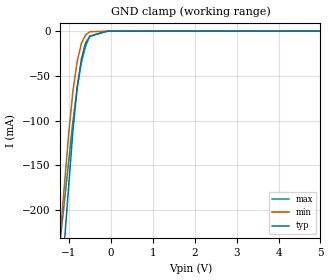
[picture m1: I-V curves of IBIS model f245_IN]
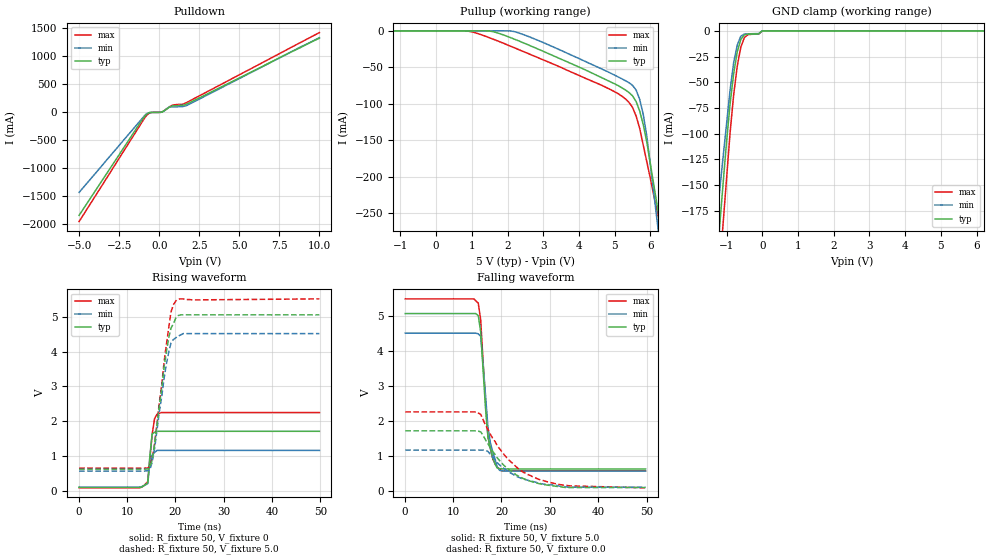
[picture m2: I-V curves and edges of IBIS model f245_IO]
| TEXAS INSTRUMENTS INCORPORATED
| Standard Linear and Logic Group
| IBIS Model of SN74F245
| OCTAL BUS TRANSCEIVERS WITH 3-STATE OUTPUTS
| SOIC 20-pin (DW), SOP 20-pin (NS), SSOP 20-pin (DB), P-DIP 20-pin (N)
[IBIS Ver]   3.2
[Comment Char]  |_char
[File Name]   sn74f245.ibs
[File Rev]   2.1 I_die
[Date]   Nov. 04, 2004
[Source]   File originated at Texas Instruments, Inc.
[Notes]   The following is a sample IBIS file for the F245.
   - FILE REV HISTORY
   - 2.1 Re-Release IBIS file on 11/05/04
   - Power-clamp data deleted as there is no power-clamp diode.
|   - All test data contained in this file are derived from
|   actual measurements.
|   - File created by Nobuhisa Ohtsubo, SLL Product Engineering.
[Disclaimer] Property of Texas Instruments Incorporated.  Unauthorized
   reproduction and/or distribution is strictly prohibited.
   This product is protected under copyright law.
   Created 2000, (C) Copyright 2000, Texas Instruments Inc.,
   All Rights Reserved.
   UNLESS THERE IS A SIGNED, WRITTEN AGREEMENT TO THE
   CONTRARY, TEXAS INSTRUMENTS () IS PROVIDING THE IBIS
   MODELS  AND WITHOUT ANY WARRANTY, EXPRESSED OR
   IMPLIED.  TI assumes no liability for:
   1) the accuracy of the IBIS models provided to your
   company;
   2) the proper functioning of these IBIS Models in your
   design or for any resulting applications; or
   3) infringement of patents, copyrights or intellectual
   property rights resulting from your use of these IBIS
   models.
   TI provides IBIS Models as a service to our customers.
   You and your company shall not distribute, sell or give
   these models to anyone else without prior written
   permission from TI.
   TI reserves the right to make changes to our products or
   to discontinue any semiconductor product or service
   without notice, and advises our customers to obtain the
   latest version of relevant information to verify, before
   placing orders, that the information being relied on is
   current.
   Please be aware that your receipt and use of the IBIS
   information provided shall serve as acceptance of these
   terms and conditions.  If you do not accept these terms,
   you should return or destroy the IBIS models and any
   other accompanying information immediately.
|   Component F245_DW
[Component]   f245_DW
[Manufacturer]  Texas Instruments, Inc.
[Package]
|   typ   min   max
R_pkg   0.038   0.033   0.045
L_pkg   5.012nH   4.110nH   6.349nH
C_pkg   0.717pF   0.530pF   0.868pF
[Pin]   signal_name   model_name   R_pin   L_pin   C_pin
1   DIR   f245_IN   0.058   5.115nH   0.725pF
2   A1   f245_IO   0.053   4.591nH   0.724pF
3   A2   f245_IO   0.049   3.754nH   0.572pF
4   A3   f245_IO   0.029   2.549nH   0.388pF
5   A4   f245_IO   0.031   2.317nH   0.316pF
6   A5   f245_IO   0.031   2.317nH   0.316pF
7   A6   f245_IO   0.029   2.556nH   0.399pF
8   A7   f245_IO   0.049   3.754nH   0.579pF
9   A8   f245_IO   0.053   4.591nH   0.724pF
10   GND   GND   0.058   5.115nH   0.725pF
11   B8   f245_IO   0.058   5.115nH   0.725pF
12   B7   f245_IO   0.053   4.591nH   0.724pF
13   B6   f245_IO   0.049   3.754nH   0.579pF
14   B5   f245_IO   0.029   2.557nH   0.399pF
15   B4   f245_IO   0.031   2.317nH   0.316pF
16   B3   f245_IO   0.031   2.317nH   0.316pF
17   B2   f245_IO   0.029   2.557nH   0.399pF
18   B1   f245_IO   0.049   3.754nH   0.579pF
19   OE_NOT   f245_IN   0.053   4.591nH   0.724pF
20   VCC   POWER   0.058   5.115nH   0.725pF
|   Component F245_NS
[Component]   f245_NS
[Manufacturer]  Texas Instruments, Inc.
[Package]
|   typ   min   max
R_pkg   0.044   0.029   0.058
L_pkg   3.666nH   2.317nH   5.115nH
C_pkg   0.548pF   0.316pF   0.725pF
[Pin]   signal_name   model_name   R_pin   L_pin   C_pin
1   DIR   f245_IN   0.058   5.115nH   0.725pF
2   A1   f245_IO   0.053   4.591nH   0.724pF
3   A2   f245_IO   0.049   3.754nH   0.572pF
4   A3   f245_IO   0.029   2.549nH   0.388pF
5   A4   f245_IO   0.031   2.317nH   0.316pF
6   A5   f245_IO   0.031   2.317nH   0.316pF
7   A6   f245_IO   0.029   2.556nH   0.399pF
8   A7   f245_IO   0.049   3.754nH   0.579pF
9   A8   f245_IO   0.053   4.591nH   0.724pF
10   GND   GND   0.058   5.115nH   0.725pF
11   B8   f245_IO   0.058   5.115nH   0.725pF
12   B7   f245_IO   0.053   4.591nH   0.724pF
13   B6   f245_IO   0.049   3.754nH   0.579pF
14   B5   f245_IO   0.029   2.557nH   0.399pF
15   B4   f245_IO   0.031   2.317nH   0.316pF
16   B3   f245_IO   0.031   2.317nH   0.316pF
17   B2   f245_IO   0.029   2.557nH   0.399pF
18   B1   f245_IO   0.049   3.754nH   0.579pF
19   OE_NOT   f245_IN   0.053   4.591nH   0.724pF
20   VCC   POWER   0.058   5.115nH   0.725pF
|   Component F245_DB
[Component]   f245_DB
[Manufacturer]  Texas Instruments, Inc.
[Package]
|   typ   min   max
R_pkg   0.040   0.035   0.051
L_pkg   3.495nH   3.035nH   4.314nH
C_pkg   0.420pF   0.346pF   0.502pF
[Pin]   signal_name   model_name   R_pin   L_pin   C_pin
1   DIR   f245_IN   0.049   4.310nH   0.502pF
2   A1   f245_IO   0.048   3.903nH   0.487pF
3   A2   f245_IO   0.035   3.189nH   0.396pF
4   A3   f245_IO   0.035   3.036nH   0.347pF
5   A4   f245_IO   0.035   3.035nH   0.367pF
6   A5   f245_IO   0.035   3.035nH   0.367pF
7   A6   f245_IO   0.035   3.036nH   0.347pF
8   A7   f245_IO   0.035   3.189nH   0.397pF
9   A8   f245_IO   0.047   3.899nH   0.488pF
10   GND   GND   0.051   4.314nH   0.500pF
11   B8   f245_IO   0.051   4.314nH   0.500pF
12   B7   f245_IO   0.047   3.899nH   0.488pF
13   B6   f245_IO   0.035   3.189nH   0.397pF
14   B5   f245_IO   0.035   3.036nH   0.346pF
15   B4   f245_IO   0.035   3.035nH   0.367pF
16   B3   f245_IO   0.035   3.035nH   0.367pF
17   B2   f245_IO   0.035   3.036nH   0.346pF
18   B1   f245_IO   0.035   3.189nH   0.397pF
19   OE_NOT   f245_IN   0.047   3.899nH   0.488pF
20   VCC   POWER   0.051   4.314nH   0.502pF
|   Component F245_N
[Component]   f245_N
[Manufacturer]   Texas Instruments, Inc.
[Package]
|   typ   min   max
R_pkg   4.300e-02   3.800e-02   5.000e-02
L_pkg   7.384e-09   4.680e-09   1.032e-08
C_pkg   5.100e-13   2.310e-13   8.210e-13
[PIN]   signal_name   model_name   R_pin   L_pin   C_pin
1   DIR   f245_IN   4.200e-02   9.427e-09   8.100e-13
2   A1   f245_IO   4.600e-02   8.544e-09   4.560e-13
3   A2   f245_IO   4.800e-02   7.163e-09   4.350e-13
4   A3   f245_IO   4.000e-02   4.825e-09   2.610e-13
5   A4   f245_IO   4.000e-02   5.284e-09   6.480e-13
6   A5   f245_IO   4.000e-02   4.686e-09   2.320e-13
7   A6   f245_IO   4.000e-02   6.359e-09   4.890e-13
8   A7   f245_IO   3.800e-02   7.982e-09   4.750e-13
9   A8   f245_IO   4.300e-02   9.403e-09   4.750e-13
10   GND   GND   5.000e-02   1.032e-08   8.050e-13
11   B8   f245_IO   5.000e-02   1.028e-08   8.100e-13
12   B7   f245_IO   4.300e-02   9.383e-09   4.770e-13
13   B6   f245_IO   3.800e-02   7.978e-09   4.760e-13
14   B5   f245_IO   4.000e-02   6.302e-09   4.920e-13
15   B4   f245_IO   4.000e-02   4.680e-09   2.310e-13
16   B3   f245_IO   4.000e-02   5.284e-09   6.480e-13
17   B2   f245_IO   4.000e-02   4.822e-09   2.610e-13
18   B1   f245_IO   4.700e-02   7.118e-09   4.390e-13
19   OE_NOT   f245_IN   4.600e-02   8.492e-09   4.610e-13
20   VCC   POWER   4.300e-02   9.348e-09   8.210e-13
| Models and submodels in the file (2): f245_IN (Input), f245_IO (I/O)
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|   Model f245_IN
[Model]   f245_IN
Model_type  Input
Polarity   Inverting
Vinl = 0.8
Vinh = 2.0
| variable   typ   min   max
C_comp   1.33pf   1.00pf   1.66pf
[Temperature Range]   25   0   70
[Voltage Range]   5.0   4.5   5.5
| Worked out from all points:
|   GND clamp passes 1 mA (typ) near -0.15 V on its own axis
[GND Clamp]
|   Voltage   I(typ)   I(min)   I(max)
-5V       -2.64A     -2.37A     -1.89A
-1.2V     -295mA     -226mA     -231mA
-1.1V     -233mA     -169mA     -188mA
-1V       -171mA     -113mA     -144mA
-900mV    -110mA     -66.1mA    -100mA
-800mV    -62.5mA    -33.7mA    -63.1mA
-700mV    -31.1mA    -13.7mA    -35.3mA
-600mV    -13mA      -4.5mA     -16.7mA
-500mV    -5.94mA    -726uA     -5.52mA
-100mV    -228uA     -140uA     -318uA
0V        -71.8uA    -105uA     -121uA
5V        68.3nA     588pA      1.05uA
|   Model f245_OUT
[Model]   f245_IO
Model_type  I/O
Polarity   Non-Inverting
Enable   Active-Low
Vinl = 0.8
Vinh = 2.0
Vmeas = 2.5v
Cref = 0pf
| variable   typ   min   max
C_comp   5.8pf   4.35pf   7.25pf
[Temperature Range]   25   0   70
[Voltage Range]   5.0   4.5   5.5
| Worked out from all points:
|   slope of the pulldown table from 0 to 0.75 V, typ, clamps not added: 6.86 ohm
|   rising waveform, R_fixture 50, V_fixture 0: 20-80 % time 618ps typ, 672ps min, 953ps max; typ from 0.093 V to 1.71 V
|   falling waveform, R_fixture 50, V_fixture 5.0: 20-80 % time 1.38ns typ, 1.6ns min, 1.34ns max; typ from 5.06 V to 0.621 V
|   rising waveform, R_fixture 50, V_fixture 5.0: 20-80 % time 2.5ns typ, 2.43ns min, 2.55ns max; typ from 0.622 V to 5.06 V
|   falling waveform, R_fixture 50, V_fixture 0.0: 20-80 % time 6.58ns typ, 6.85ns min, 7.83ns max; typ from 1.71 V to 0.09 V
[Pulldown]
|   Voltage   I(typ)   I(min)   I(max)
-5V       -1.84A     -1.43A     -1.95A
-1.1V     -150mA     -124mA     -189mA
-900mV    -70.8mA    -57.2mA    -98.7mA
-700mV    -20.4mA    -13.9mA    -34.2mA
-500mV    -3.88mA    -3.11mA    -6.51mA
100mV     -1.74mA    -1.96mA    -1.08mA
200mV     6.05mA     4.34mA     8.27mA
600mV     83.5mA     85.4mA     87.7mA
900mV     114mA      94.8mA     131mA
1.4V      122mA      99.3mA     141mA
1.7V      144mA      117mA      170mA
10V       1.32A      1.33A      1.42A
[Pullup]
|   Voltage   II(typ)   I(min)   I(max)
-5V       214nA      3.02nA     463nA
800mV     -2.09uA    1.93nA     -65.5uA
1.6V      -1.21mA    -6.69uA    -11.5mA
2.4V      -15.6mA    -4.37mA    -27.5mA
5.1V      -75.2mA    -63.3mA    -86.3mA
5.4V      -84.6mA    -71.1mA    -98.2mA
5.6V      -97.1mA    -81.3mA    -117mA
5.8V      -129mA     -115mA     -157mA
5.9V      -153mA     -145mA     -180mA
6.2V      -243mA     -266mA     -250mA
6.3V      -273mA     -306mA     -273mA
10V       -1.38A     -1.8A      -1.13A
[GND Clamp]
|   Voltage   I(typ)   I(min)   I(max)
-5V       -1.84A     -1.43A     -1.95A
-1.3V     -237mA     -191mA     -279mA
-1.2V     -193mA     -158mA     -234mA
-1.1V     -150mA     -124mA     -189mA
-1V       -108mA     -90.6mA    -144mA
-900mV    -70.8mA    -57.2mA    -98.7mA
-800mV    -41.5mA    -30.7mA    -62mA
-700mV    -20.4mA    -13.9mA    -34.2mA
-600mV    -8.33mA    -5.17mA    -15.8mA
-500mV    -3.88mA    -3.11mA    -6.51mA
0V        2.8uA      2.55uA     2.91uA
10V       2.8uA      2.55uA     2.91uA
[Ramp]
| variable   typ   min   max
dV/dt_r   1.230/0.904n   1.020/0.797n   1.428/1.119n
dV/dt_f   2.844/1.449n   2.526/1.698n   3.030/1.376n
R_load = 50
[Rising Waveform]
R_fixture = 50
V_fixture = 0
|   Time   V(typ)   V(min)   V(max)
97.7ps    92.9mV     104mV      83.6mV
12.3ns    94.5mV     103mV      83.6mV
13.8ns    173mV      166mV      189mV
14.3ns    228mV      206mV      260mV
14.7ns    937mV      757mV      859mV
15.2ns    1.63V      1.03V      1.61V
15.7ns    1.68V      1.1V       2.07V
16.2ns    1.71V      1.16V      2.2V
16.7ns    1.71V      1.16V      2.23V
49.8ns    1.71V      1.16V      2.25V
[Falling Waveform]
R_fixture = 50
V_fixture = 5.0
V_fixture_min = 4.5
V_fixture_max = 5.5
|   Time   V(typ)   V(min)   V(max)
97.7ps    5.06V      4.5V       5.48V
14.3ns    5.06V      4.5V       5.48V
15.2ns    5V         4.48V      5.36V
15.7ns    4.54V      4.41V      4.88V
16.7ns    2.35V      2.72V      2.57V
17.2ns    1.54V      1.81V      1.55V
17.7ns    1.21V      1.37V      1.21V
18.7ns    754mV      884mV      763mV
20.1ns    624mV      568mV      565mV
49.8ns    621mV      560mV      565mV
[Rising Waveform]
R_fixture = 50
V_fixture = 5.0
V_fixture_min = 4.5
V_fixture_max = 5.5
|   Time   V(typ)   V(min)   V(max)
97.7ps    622mV      566mV      651mV
14.7ns    654mV      595mV      707mV
15.2ns    886mV      816mV      906mV
15.7ns    1.33V      1.21V      1.33V
17.7ns    3.59V      3.26V      3.73V
18.7ns    4.44V      4.03V      4.75V
19.1ns    4.68V      4.25V      5.14V
19.6ns    4.8V       4.35V      5.35V
20.6ns    5.04V      4.45V      5.51V
49.8ns    5.06V      4.52V      5.52V
[Falling Waveform]
R_fixture = 50
V_fixture = 0.0
|   Time   V(typ)   V(min)   V(max)
97.7ps    1.71V      1.16V      2.25V
15.2ns    1.7V       1.16V      2.22V
15.7ns    1.68V      1.16V      2.18V
17.2ns    1.34V      1.12V      1.75V
19.1ns    942mV      802mV      1.29V
21.1ns    657mV      581mV      940mV
24.5ns    346mV      331mV      526mV
27.9ns    198mV      209mV      315mV
34.3ns    90.6mV     100mV      135mV
49.8ns    90.1mV     100mV      81mV
